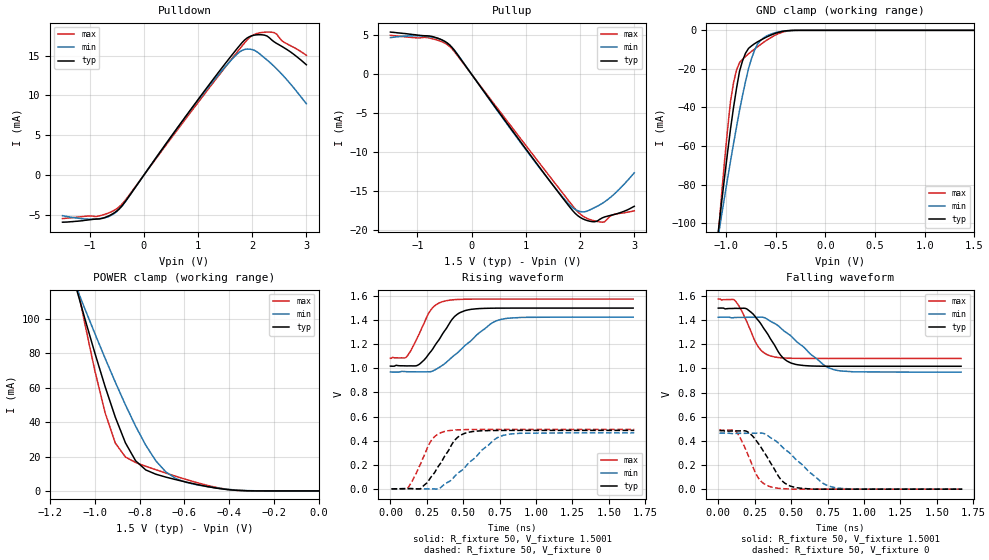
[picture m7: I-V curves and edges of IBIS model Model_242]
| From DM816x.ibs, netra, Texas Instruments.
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| Model based on original model for BSHTLTCSCDDVGPBFZ
|   Sub model SLOWEST_4MA_5PER_P_1P5
[model]   Model_242
|[Description]  1.5V-3-STATE-X-SLOWEST, 4MA, +-5%
|[Input Load]
|[Output Drive] SLOWEST, 4MA
|Voltage   1.5V
|Mode   3-STATE
Model_type   3-state
Polarity   Non-Inverting
Enable   Active-Low
Cref =  15.0000pF
Rref =  100.0000M
Vref =  0V
Vmeas =  0.75005
C_comp   1.5249p   1.4275p   1.6205p
[Model Spec]
[Temperature Range]   25   125   -40
[Voltage Range]   1.5   1.425   1.575
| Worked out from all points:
|   slope of the pulldown table from 0 to 0.225 V, typ, clamps not added: 103 ohm
|   slope of the pullup table from 0 to 0.225 V, typ, clamps not added: 103 ohm
|   GND clamp passes 1 mA (typ) near -0.47 V on its own axis
|   POWER clamp passes 1 mA (typ) near -0.42 V on its own axis
|   rising waveform, R_fixture 50, V_fixture 1.5001: 20-80 % time 161ps typ, 259ps min, 118ps max; typ from 1.02 V to 1.5 V
|   rising waveform, R_fixture 50, V_fixture 0: 20-80 % time 154ps typ, 248ps min, 113ps max; typ from 0 V to 0.485 V
|   falling waveform, R_fixture 50, V_fixture 1.5001: 20-80 % time 155ps typ, 264ps min, 113ps max; typ from 1.5 V to 1.02 V
|   falling waveform, R_fixture 50, V_fixture 0: 20-80 % time 150ps typ, 254ps min, 109ps max; typ from 0.485 V to 0 V
[POWER_clamp]
-1.5V     321.7mA    260.6mA    415.9mA
-1.076V   114.2mA    115.8mA    116.9mA
-1.061V   107.2mA    110.9mA    107.1mA
-954.6mV  60.59mA    77.06mA    45.35mA
-909.2mV  42.85mA    63.21mA    27.81mA
-863.7mV  27.9mA     49.99mA    19.69mA
-818.2mV  17.49mA    37.63mA    16.52mA
-772.8mV  12.19mA    26.53mA    14.33mA
-681.9mV  7.985mA    10.89mA    10.33mA
-590.9mV  5.094mA    4.955mA    6.6mA
-363.7mV  298.5uA    465.2uA    297.6uA
0V        1.518nA    24.08nA    367.8pA
[Pulldown]
-1.5V     -5.88mA    -5.06mA    -5.43mA
-863.7mV  -5.487mA   -5.465mA   -5.158mA
-500mV    -4.487mA   -4.559mA   -4.195mA
-318.2mV  -3.078mA   -3.107mA   -2.93mA
1.046V    9.891mA    9.776mA    9.509mA
1.591V    14.76mA    14.27mA    14.3mA
1.818V    16.65mA    15.66mA    16.24mA
1.955V    17.39mA    15.81mA    17.28mA
2.091V    17.61mA    15.47mA    17.77mA
2.273V    17.46mA    14.46mA    17.94mA
2.364V    16.94mA    13.92mA    17.92mA
3V        13.85mA    8.96mA     15.04mA
[Pullup]
-1.5V     5.43mA     4.72mA     5.02mA
-818.2mV  4.951mA    4.862mA    4.719mA
-590.9mV  4.551mA    4.546mA    4.297mA
-409.1mV  3.79mA     3.793mA    3.605mA
1.227V    -11.69mA   -11.75mA   -11.17mA
1.727V    -16.29mA   -16.13mA   -15.66mA
1.909V    -17.82mA   -17.32mA   -17.25mA
2.046V    -18.51mA   -17.64mA   -18.15mA
2.227V    -18.89mA   -17.22mA   -18.72mA
2.409V    -18.41mA   -16.55mA   -18.96mA
2.591V    -18.04mA   -15.6mA    -18.04mA
3V        -16.92mA   -12.63mA   -17.5mA
[GND_clamp]
-1.5V     -310.1mA   -250.5mA   -402.5mA
-1.076V   -103.6mA   -106.2mA   -105.2mA
-1.046V   -89.81mA   -96.36mA   -86.02mA
-954.6mV  -51.22mA   -67.87mA   -36.88mA
-924.3mV  -40.08mA   -58.86mA   -27.29mA
-863.7mV  -21.24mA   -41.56mA   -16.73mA
-833.4mV  -15.8mA    -33.75mA   -15.03mA
-772.8mV  -9.345mA   -19.75mA   -12.19mA
-712.2mV  -6.928mA   -10.35mA   -9.704mA
-621.3mV  -4.261mA   -3.896mA   -6.225mA
-409.1mV  -337.1uA   -289.1uA   -618.9uA
1.5V      1.518nA    257.2nA    299pA
[Ramp]
dV/dt_f   0.38592/0.22813884n   0.364576/0.36618276n   0.39392/0.17398082n
dV/dt_r 0.38901696/0.22246991n  0.3735784/0.34641548n 0.39462003/0.17160524n
R_load = 50
[Rising Waveform]
R_fixture = 50
V_fixture = 1.5001
V_fixture_min = 1.425
V_fixture_max = 1.575
0s        1.018V     969.9mV    1.083V
109.2ps   1.02V      972.5mV    1.093V
197.9ps   1.033V     970.9mV    1.286V
282.2ps   1.147V     974.5mV    1.492V
371.8ps   1.31V      1.038V     1.558V
424.5ps   1.408V     1.094V     1.568V
478.8ps   1.463V     1.15V      1.572V
684.2ps   1.499V     1.365V     1.575V
758.8ps   1.5V       1.406V     1.575V
1.667ns   1.5V       1.425V     1.575V
[Rising Waveform]
R_fixture = 50
V_fixture = 0
V_fixture_min = 0
V_fixture_max = 0
7.64ps    0V         0V         0V
114.6ps   2.3mV      2.804mV    0V
205.3ps   0V         0V         202.4mV
283.2ps   104.8mV    0V         405.6mV
368.6ps   263.4mV    35.87mV    475.3mV
438.9ps   399.5mV    100.9mV    488.1mV
495.8ps   453.8mV    158.9mV    491.3mV
634.8ps   482.4mV    328.3mV    493mV
772.9ps   485.1mV    443.6mV    493.2mV
1.674ns   485.4mV    464.7mV    493.2mV
[Falling Waveform]
R_fixture = 50
V_fixture = 1.5001
V_fixture_min = 1.425
V_fixture_max = 1.575
0s        1.5V       1.424V     1.575V
113.5ps   1.497V     1.421V     1.564V
194.3ps   1.494V     1.423V     1.391V
277.8ps   1.393V     1.424V     1.173V
365ps     1.232V     1.386V     1.101V
427.9ps   1.11V      1.335V     1.088V
502.7ps   1.043V     1.265V     1.084V
722.2ps   1.018V     1.03V      1.083V
792.7ps   1.018V     989.6mV    1.083V
1.667ns   1.018V     969.4mV    1.083V
[Falling Waveform]
R_fixture = 50
V_fixture = 0
V_fixture_min = 0
V_fixture_max = 0
7.64ps    484.8mV    463.8mV    492.3mV
121.8ps   482.8mV    461.6mV    477.1mV
203ps     473.6mV    463.2mV    286.7mV
280.4ps   369.4mV    464.1mV    83.9mV
365ps     205.4mV    421.3mV    17.44mV
432.2ps   76.7mV     357.8mV    5.131mV
493.6ps   25.82mV    295.8mV    0V
628.6ps   2.631mV    137.9mV    0V
761.1ps   0V         24.51mV    0V
1.674ns   0V         0V         0V
